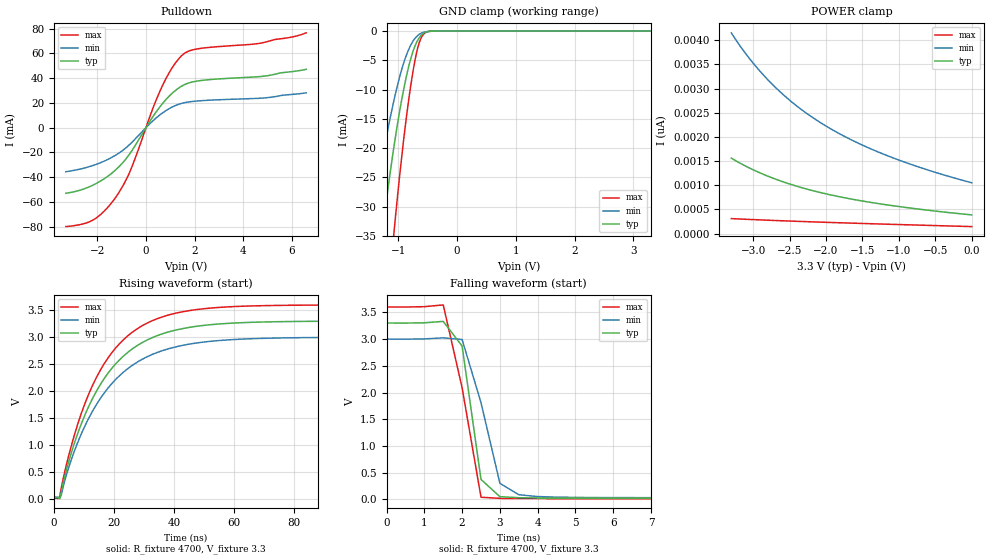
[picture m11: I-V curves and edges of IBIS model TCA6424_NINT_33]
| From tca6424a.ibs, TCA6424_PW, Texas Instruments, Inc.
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[Model]   TCA6424_NINT_33
Model_type  Open_drain
Enable   Active-Low
Vref =   3.3
Rref =   4700
Cref =   50p
Vmeas =   1.65
| variable   typ   min   max
C_comp   2.33pF   1.87pF   2.53pF
| C_pulldown   3.17pF   2.31pF   3.96pF
| C_tri-state   2.33pF   1.87pF   2.53pF
[Temperature Range]   40   100   -40
| Ambient temperature   25   85   -40
[Voltage range]   3.3   3   3.6
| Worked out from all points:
|   slope of the pulldown table from 0 to 0.495 V, typ, clamps not added: 33.5 ohm
|   GND clamp passes 1 mA (typ) near -0.63 V on its own axis
|   rising waveform, R_fixture 4700, V_fixture 3.3: 20-80 % time 18.2ns typ, 19.2ns min, 17.3ns max; typ from 0.021 V to 3.3 V
|   falling waveform, R_fixture 4700, V_fixture 3.3: 20-80 % time 394ps typ, 645ps min, 588ps max; typ from 3.3 V to 0.021 V
[GND Clamp]
| TCA6424_NINT_33
|   Voltage   I(typ)   I(min)   I(max)
-3.3V     -260.7mA   -193.9mA   -362.2mA
-1.47V    -51.46mA   -34.11mA   -82.14mA
-1.28V    -35.02mA   -22.38mA   -57.9mA
-1.25V    -32.61mA   -20.69mA   -54.27mA
-1.08V    -20.12mA   -12.09mA   -35.04mA
-1.055V   -18.47mA   -10.98mA   -32.43mA
-930mV    -11.07mA   -6.159mA   -20.39mA
-800mV    -5.162mA   -2.633mA   -10.11mA
-700mV    -2.172mA   -1.062mA   -4.18mA
-615mV    -769.4uA   -394.8uA   -1.247mA
-410mV    -15.75uA   -12.96uA   -12.82uA
3.3V      385.2pA    1.176nA    131.1pA
[POWER Clamp]
| TCA6424_NINT_33
|   Voltage   I(typ)   I(min)   I(max)
-3.3V     1.563nA    4.154nA    308.9pA
-3.18V    1.456nA    3.882nA    300.3pA
-3.035V   1.344nA    3.591nA    290.4pA
-2.89V    1.244nA    3.332nA    281pA
-2.74V    1.152nA    3.092nA    271.8pA
-2.585V   1.068nA    2.871nA    262.8pA
-2.42V    987.5pA    2.662nA    253.6pA
-2.06V    842.1pA    2.28nA     234.8pA
-1.65V    712.9pA    1.937nA    215pA
-1.18V    596.6pA    1.624nA    193.6pA
-625mV    486.6pA    1.326nA    169.6pA
-48.03fV  385.2pA    1.05nA     143.4pA
[Pulldown]
| TCA6424_NINT_33
|   Voltage   I(typ)   I(min)   I(max)
-3.3V     -52.99mA   -35.6mA    -79.91mA
-2.15V    -46.11mA   -30.34mA   -74.26mA
-1.685V   -40.79mA   -26.72mA   -66.72mA
-1.22V    -33.58mA   -21.85mA   -55.5mA
-630mV    -20.06mA   -12.81mA   -34.11mA
255mV     8.017mA    4.951mA    14.05mA
670mV     19.21mA    11.72mA    33.54mA
1.115V    28.43mA    17.02mA    49.47mA
1.535V    34.24mA    19.97mA    59.3mA
2.105V    37.65mA    21.54mA    63.61mA
4.625V    41.18mA    23.71mA    67.98mA
6.6V      47.17mA    28.14mA    76.63mA
[Ramp]
| TCA6424_NINT_33
| variable   typ   min   max
dV/dt_r   1.98/1.82E-08   1.79/1.92E-08   2.17/1.73E-08
dV/dt_f   2.00/3.69E-10   1.81/5.16E-10   2.18/2.74E-10
R_load = 4700
[Rising Waveform]
| TCA6424_NINT_33
R_fixture =   4700
C_fixture =   0
L_fixture =   0
V_fixture =   3.3
V_fixture_min = 3
V_fixture_max = 3.6
|   Time   V(typ)   V(min)   V(max)
0s        21.2mV     30.98mV    13.17mV
2ns       1.394mV    15.31mV    49.99mV
6ns       885.1mV    755.1mV    1.019V
11ns      1.64V      1.427V     1.861V
19ns      2.401V     2.119V     2.69V
24.5ns    2.713V     2.412V     3.02V
31ns      2.947V     2.636V     3.261V
48ns      3.207V     2.897V     3.517V
96ns      3.298V     2.997V     3.599V
520ns     3.3V       3V         3.6V
[Falling Waveform]
| TCA6424_NINT_33
R_fixture =   4700
C_fixture =   0
L_fixture =   0
V_fixture =   3.3
V_fixture_min = 3
V_fixture_max = 3.6
|   Time   V(typ)   V(min)   V(max)
0s        3.3V       3V         3.6V
1ns       3.304V     3.002V     3.606V
1.5ns     3.33V      3.023V     3.639V
2ns       2.869V     2.991V     2.087V
2.5ns     373.5mV    1.809V     40.45mV
3ns       51.09mV    300.3mV    19.52mV
3.5ns     31.42mV    87.68mV    16.15mV
4ns       26.28mV    53.13mV    14.78mV
7.5ns     21.49mV    31.91mV    13.27mV
520ns     21.2mV     30.98mV    13.17mV
